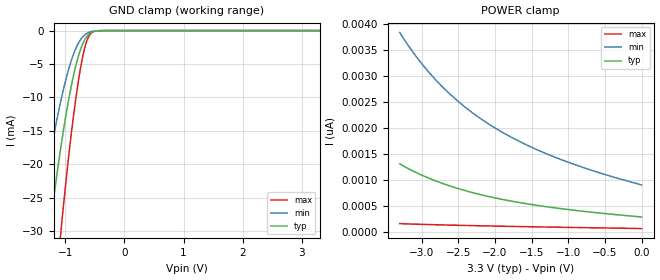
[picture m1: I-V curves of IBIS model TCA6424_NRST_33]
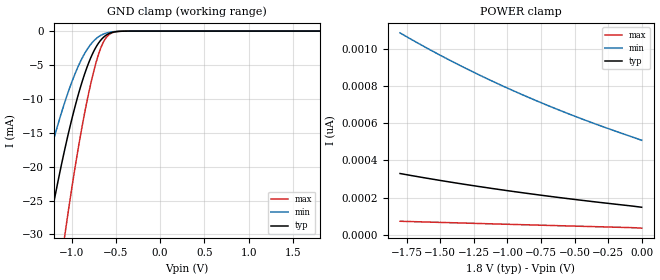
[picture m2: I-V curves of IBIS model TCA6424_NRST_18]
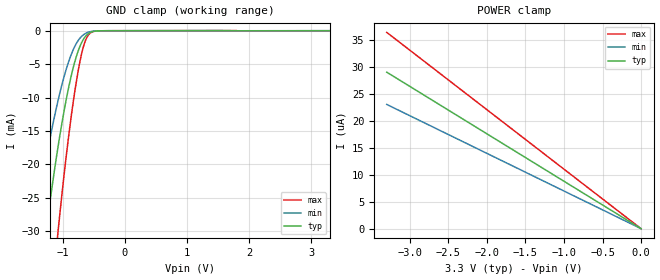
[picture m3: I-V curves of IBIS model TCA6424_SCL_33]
| TEXAS INSTRUMENTS INCORPORATED
| Standard Linear and Logic Group
| IBIS Model of TCA6424
| LOW-VOLTAGE 24-BIT I2C AND SMBus I/O EXPANDER WITH INTERRUPT OUTPUT,
| RESET, AND CONFIGURATION REGISTERS
| This file contains package information for the following:
|  QFN 32-pin (RGJ) package as [Component] TCA6424_RGJ
| This device can be powered at the following Vccs:
|  5 volt Vcc
|  3.3 volt Vcc
|  2.5 volt Vcc
|  1.8 volt Vcc
| This file provides unique models under the [Model Selector] for each Vcc.
| For operation at a specific Vcc, select the appropriate model after each
| [Model Selector] keyword.
[IBIS Ver]   3.2
[Comment char]  |_char
[File Name]   tca6424a.ibs
[File Rev]   1.0 | x_die
[Date]   July 13, 2009
[Source]   Data created from TI-SPICE simulations at TI-SLL.
[Notes]   The following is an IBIS list for the TCA6424.
   Please contact sllibis@ti.com with questions and
   comments concerning SLL IBIS models.
[Disclaimer] Property of Texas Instruments Incorporated.  Unauthorized
   reproduction and/or distribution is strictly prohibited.
   This product is protected under copyright law.
   Created  2008, (C) Copyright  2008, Texas Instruments
   Incorporated, All Rights Reserved
   UNLESS THERE IS A SIGNED, WRITTEN AGREEMENT TO THE
   CONTRARY, TEXAS INSTRUMENTS (TI) IS PROVIDING THE IBIS
   MODELS  AND WITHOUT ANY WARRANTY, EXPRESSED OR
   IMPLIED.  TI assumes no liability for:
   1) the accuracy of the IBIS models provided to your
   company;
   2) the proper functioning of these IBIS Models in your
   design or for any resulting applications; or
   3) infringement of patents, copyrights or intellectual
   property rights resulting from your use of these IBIS
   models.
   TI provides IBIS Models as a service to our customers.
   You and your company shall not distribute, sell or give
   these models to anyone else without prior written
   permission from TI.
   TI reserves the right to make changes to our products or
   to discontinue any semiconductor product or service
   without notice, and advises our customers to obtain the
   latest version of relevant information to verify, before
   placing orders, that the information being relied on is
   current.
   Please be aware that your receipt and use of the IBIS
   information provided shall serve as acceptance of these
   terms and conditions.  If you do not accept these terms,
   you should return or destroy the IBIS models and any
   other accompanying information immediately.
| Component TCA6424_RGJ 32-PIN QFN
[Component]   TCA6424_PW
[Manufacturer]   Texas Instruments, Inc.
[Package]
|   typ   min   max
R_pkg   4.500e-02   3.800e-02   5.100e-02
L_pkg   2.593e-09   2.447e-09   3.080e-09
C_pkg   2.810e-13   2.430e-13   3.770e-13
[Pin]   signal_name   model_name   R_pin   L_pin   C_pin
1   P00   TCA6424_P   5.100e-02   2.447e-09   2.430e-13
2   P01   TCA6424_P   5.100e-02   2.447e-09   2.430e-13
3   P02   TCA6424_P   5.100e-02   2.512e-09   2.550e-13
4   P03   TCA6424_P   3.800e-02   2.458e-09   2.810e-13
5   P04   TCA6424_P   3.900e-02   2.832e-09   3.160e-13
6   P05   TCA6424_P   3.800e-02   2.460e-09   2.790e-13
7   P06   TCA6424_P   5.100e-02   2.512e-09   2.550e-13
8   P07   TCA6424_P   5.100e-02   2.447e-09   2.430e-13
9   P10   TCA6424_P   5.100e-02   2.447e-09   2.430e-13
10   P11   TCA6424_P   5.100e-02   2.447e-09   2.430e-13
11   P12   TCA6424_P   5.100e-02   2.512e-09   2.550e-13
12   P13   TCA6424_P   3.800e-02   2.458e-09   2.810e-13
13   P14   TCA6424_P   3.900e-02   2.832e-09   3.160e-13
14   P15   TCA6424_P   3.800e-02   2.460e-09   2.790e-13
15   P16   TCA6424_P   5.100e-02   2.512e-09   2.550e-13
16   P17   TCA6424_P   5.100e-02   2.447e-09   2.430e-13
17   P20   TCA6424_P   5.100e-02   2.447e-09   2.430e-13
18   P21   TCA6424_P   5.100e-02   2.447e-09   2.430e-13
19   P22   TCA6424_P   5.100e-02   2.512e-09   2.550e-13
20   P23   TCA6424_P   3.800e-02   2.458e-09   2.810e-13
21   P24   TCA6424_P   3.900e-02   2.832e-09   3.160e-13
22   P25   TCA6424_P   3.800e-02   2.460e-09   2.790e-13
23   P26   TCA6424_P   5.100e-02   2.512e-09   2.550e-13
24   P27   TCA6424_P   5.100e-02   2.447e-09   2.430e-13
25   GND   GND   4.000e-02   3.080e-09   3.770e-13
26   ADDR   TCA6424_ADDR   3.800e-02   2.458e-09   2.810e-13
27   VCCP   POWER   3.900e-02   2.832e-09   3.160e-13
28   NRESET   TCA6424_NRST   5.100e-02   2.512e-09   2.550e-13
29   SCL   TCA6424_SCL   5.100e-02   2.512e-09   2.550e-13
30   SDA   TCA6424_SDA   3.800e-02   2.459e-09   2.790e-13
31   VCCI   POWER   4.000e-02   3.080e-09   3.770e-13
32   NINT   TCA6424_NINT   5.100e-02   2.447e-09   2.430e-13
| Model TCA6424_NRST
[Model Selector]   TCA6424_NRST
TCA6424_NRST_50   5 volt Vcc
TCA6424_NRST_33   3.3 volt Vcc
TCA6424_NRST_25   2.5 volt Vcc
TCA6424_NRST_18   1.8 volt Vcc
| Model TCA6424_SCL
[Model Selector]   TCA6424_SCL
TCA6424_SCL_50   5 volt Vcc
TCA6424_SCL_33   3.3 volt Vcc
TCA6424_SCL_25   2.5 volt Vcc
TCA6424_SCL_18   1.8 volt Vcc
| Model TCA6424_ADDR
[Model Selector]   TCA6424_ADDR
TCA6424_ADDR_50   5 volt Vcc
TCA6424_ADDR_33   3.3 volt Vcc
TCA6424_ADDR_25   2.5 volt Vcc
TCA6424_ADDR_18   1.8 volt Vcc
| Model TCA6424_P
[Model Selector]   TCA6424_P
TCA6424_P_50   5 volt Vcc
TCA6424_P_33   3.3 volt Vcc
TCA6424_P_25   2.5 volt Vcc
TCA6424_P_18   1.8 volt Vcc
| Model TCA6424_SDA
[Model Selector]   TCA6424_SDA
TCA6424_SDA_50   5 volt Vcc
TCA6424_SDA_33   3.3 volt Vcc
TCA6424_SDA_25   2.5 volt Vcc
TCA6424_SDA_18   1.8 volt Vcc
| Model TCA6424_NINT
[Model Selector]   TCA6424_NINT
TCA6424_NINT_50   5 volt Vcc
TCA6424_NINT_33   3.3 volt Vcc
TCA6424_NINT_25   2.5 volt Vcc
TCA6424_NINT_18   1.8 volt Vcc
| Models and submodels in the file (24): TCA6424_NRST_50 (Input), TCA6424_NRST_33 (Input), TCA6424_NRST_25 (Input), TCA6424_NRST_18 (Input), TCA6424_SCL_50 (Input), TCA6424_SCL_33 (Input), TCA6424_SCL_25 (Input), TCA6424_SCL_18 (Input), TCA6424_ADDR_50 (Input), TCA6424_ADDR_33 (Input), TCA6424_ADDR_25 (Input), TCA6424_ADDR_18 (Input), TCA6424_P_50 (I/O), TCA6424_P_33 (I/O), TCA6424_P_25 (I/O), TCA6424_P_18 (I/O), TCA6424_SDA_50 (I/O_open_drain), TCA6424_SDA_33 (I/O_open_drain), TCA6424_SDA_25 (I/O_open_drain), TCA6424_SDA_18 (I/O_open_drain), TCA6424_NINT_50 (Open_drain), TCA6424_NINT_33 (Open_drain), TCA6424_NINT_25 (Open_drain), TCA6424_NINT_18 (Open_drain)
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[Model]   TCA6424_NRST_33
Model_type  Input
Vinl=0.9
Vinh=2.52
| variable   typ   min   max
C_comp   2.22pF   1.76pF   2.42pF
[Temperature Range]   40   100   -40
| Ambient temperature   25   85   -40
[Voltage range]   3.3   3   3.6
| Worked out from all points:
|   GND clamp passes 1 mA (typ) near -0.65 V on its own axis
[GND Clamp]
| TCA6424_NRST_33
|   Voltage   I(typ)   I(min)   I(max)
-3.3V     -229.8mA   -173.1mA   -314.8mA
-1.49V    -47mA      -31.57mA   -73.96mA
-1.455V   -44.17mA   -29.5mA    -69.9mA
-1.285V   -31.19mA   -20.13mA   -51.01mA
-1.255V   -29.05mA   -18.6mA    -47.84mA
-1.08V    -17.66mA   -10.65mA   -30.52mA
-945mV    -10.37mA   -5.81mA    -18.9mA
-810mV    -4.799mA   -2.428mA   -9.366mA
-700mV    -1.861mA   -882.4uA   -3.61mA
-615mV    -655uA     -320.4uA   -1.07mA
-410mV    -13.36uA   -10.66uA   -11.01uA
3.3V      289.3pA    1.025nA    57.78pA
[POWER Clamp]
| TCA6424_NRST_33
|   Voltage   I(typ)   I(min)   I(max)
-3.3V     1.315nA    3.842nA    162.7pA
-3.18V    1.219nA    3.582nA    157.1pA
-3.035V   1.119nA    3.303nA    150.7pA
-2.89V    1.03nA     3.055nA    144.8pA
-2.74V    948.5pA    2.827nA    139.1pA
-2.585V   873.6pA    2.616nA    133.6pA
-2.42V    803.1pA    2.417nA    128.2pA
-2.06V    676pA      2.056nA    117.3pA
-1.65V    564.5pA    1.732nA    106.3pA
-1.18V    465.7pA    1.439nA    94.89pA
-640mV    376.5pA    1.169nA    82.73pA
-48.03fV  289.3pA    907.3pA    66.29pA
[Model]   TCA6424_NRST_18
Model_type  Input
Vinl=0.495
Vinh=1.365
| variable   typ   min   max
C_comp   2.21pF   1.67pF   2.46pF
[Temperature Range]   40   100   -40
| Ambient temperature   25   85   -40
[Voltage range]   1.8   1.65   1.95
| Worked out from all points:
|   GND clamp passes 1 mA (typ) near -0.65 V on its own axis
[GND Clamp]
| TCA6424_NRST_18
|   Voltage   I(typ)   I(min)   I(max)
-1.8V     -74.02mA   -51.67mA   -111.7mA
-1.45V    -43.77mA   -29.21mA   -69.33mA
-1.27V    -30.12mA   -19.36mA   -49.42mA
-1.25V    -28.7mA    -18.35mA   -47.31mA
-1.07V    -17.07mA   -10.25mA   -29.6mA
-960mV    -11.11mA   -6.281mA   -20.1mA
-855mV    -6.438mA   -3.375mA   -12.27mA
-765mV    -3.406mA   -1.667mA   -6.757mA
-680mV    -1.498mA   -708.4uA   -2.836mA
-590mV    -450.5uA   -228.8uA   -677.8uA
-475mV    -54.97uA   -37.86uA   -56.06uA
1.8V      147.6pA    546pA      30.99pA
[POWER Clamp]
| TCA6424_NRST_18
|   Voltage   I(typ)   I(min)   I(max)
-1.8V     329.2pA    1.086nA    72.27pA
-1.605V   304.6pA    1.007nA    68.21pA
-1.385V   278.5pA    922.7pA    63.7pA
-1.17V    254.7pA    846.2pA    59.35pA
-950mV    231.9pA    773pA      54.95pA
-730mV    210.6pA    704.8pA    50.6pA
-505mV    190.2pA    639.7pA    46.2pA
-290mV    171.9pA    581.8pA    42.03pA
-16.28fV  147.6pA    508.2pA    35.04pA
[Model]   TCA6424_SCL_33
Model_type  Input
Vinl=0.9
Vinh=2.52
| variable   typ   min   max
C_comp   2.17pF   1.72pF   2.37pF
[Temperature Range]   40   100   -40
| Ambient temperature   25   85   -40
[Voltage range]   3.3   3   3.6
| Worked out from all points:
|   GND clamp passes 1 mA (typ) near -0.65 V on its own axis
[GND Clamp]
| TCA6424_SCL_33
|   Voltage   I(typ)   I(min)   I(max)
-3.3V     -229.8mA   -173.1mA   -314.8mA
-1.49V    -47.01mA   -31.58mA   -73.96mA
-1.455V   -44.17mA   -29.5mA    -69.91mA
-1.285V   -31.2mA    -20.13mA   -51.01mA
-1.255V   -29.06mA   -18.61mA   -47.84mA
-1.08V    -17.66mA   -10.65mA   -30.52mA
-945mV    -10.38mA   -5.815mA   -18.91mA
-810mV    -4.804mA   -2.432mA   -9.37mA
-700mV    -1.866mA   -886.6uA   -3.615mA
-615mV    -659.7uA   -324.3uA   -1.075mA
-400mV    -14.1uA    -11.42uA   -12.78uA
3.3V      289.3pA    2.092uA    -3.305uA
[POWER Clamp]
| TCA6424_SCL_33
|   Voltage   I(typ)   I(min)   I(max)
-3.3V     28.99uA    23.01uA    36.36uA
-2.98V    26.18uA    20.78uA    32.83uA
-1.81V    15.9uA     12.62uA    19.94uA
-48.03fV  289.3pA    907.4pA    66.29pA
